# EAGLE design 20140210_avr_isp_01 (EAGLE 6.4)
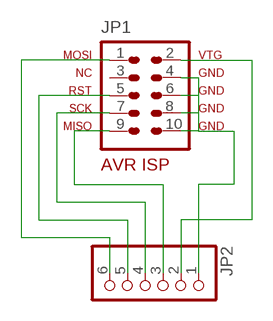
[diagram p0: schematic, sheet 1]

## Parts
JP1  AVR-ISP-10EDGE  [AVR-ISP-10-EDGE]
JP2  PINHD-1X6/90  [1X06/90]

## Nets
N$1: JP1.1 JP2.6
N$2: JP1.5 JP2.5
N$3: JP1.7 JP2.4
N$4: JP1.9 JP2.3
N$5: JP1.2 JP2.2
N$6: JP1.4 JP1.6 JP1.8 JP1.10 JP2.1
Unconnected: JP1.3

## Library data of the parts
JP1 = avr-4:AVR-ISP-10: AVR ISP-10 Serial Programming Header
JP2 = pinhead:PINHD-1X6: PIN HEADER

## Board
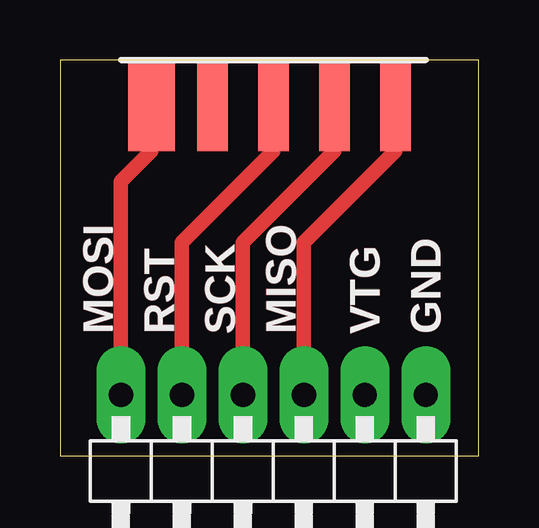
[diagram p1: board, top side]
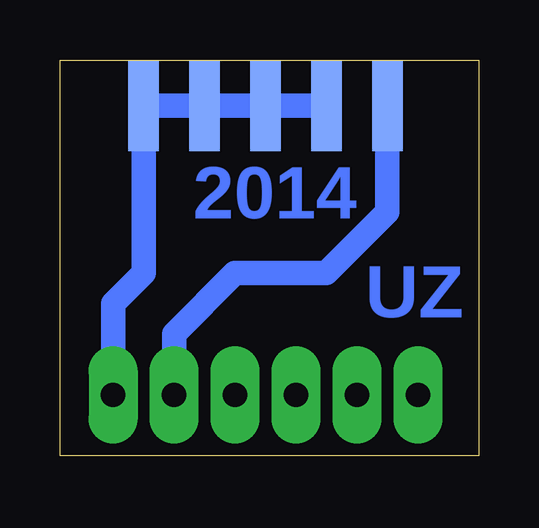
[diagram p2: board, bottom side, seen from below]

Size 17.45 x 16.5 mm. Coordinates in mm from the lower left corner, seen from the top.
Outline: 0,0 17.45,0 17.45,16.5 0,16.5 0,0
Copper layers (1*16): Top 0.035mm / dielectric 1.5mm / Bottom 0.035mm
Design rules "default *": minimum track width 10mil, minimum drill 24mil, track to track 8mil, track to pad 8mil, pad to pad 8mil, via to via 8mil, smd to smd 8mil, copper to edge 40mil, drill to drill 8mil, minimum pad ring 10mil, minimum via ring 8mil, stop-mask expansion 4mil, vias tented up to drill 0mil, thermal gap 10mil

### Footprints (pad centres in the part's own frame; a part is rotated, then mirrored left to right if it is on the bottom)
AVR-ISP-10-EDGE = smd 1.93 x 3.81: 1 -5.08,-1.905 | smd 1.27 x 3.81 bottom: 2 -5.08,-1.905; 4 -2.54,-1.905; 6 0,-1.905; 8 2.54,-1.905; 10 5.08,-1.905 | smd 1.27 x 3.81: 3 -2.54,-1.905; 5 0,-1.905; 7 2.54,-1.905; 9 5.08,-1.905
1X06/90 = drill 1.016 long: 1 -6.35,-3.81; 2 -3.81,-3.81; 3 -1.27,-3.81; 4 1.27,-3.81; 5 3.81,-3.81; 6 6.35,-3.81

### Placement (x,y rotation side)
JP1  8.89,16.51 0 top
JP2  8.89,-1.27 180 top

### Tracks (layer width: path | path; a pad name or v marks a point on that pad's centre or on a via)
N$1
  Top 0.61: JP1.1 3.81,12.7 2.54,11.43 JP2.6
N$2
  Top 0.61: JP1.5 8.89,12.7 5.08,8.89 JP2.5
N$3
  Top 0.61: JP1.7 11.43,12.7 7.62,8.89 JP2.4
N$4
  Top 0.61: JP1.9 13.97,12.7 10.16,8.89 JP2.3
N$5
  Bottom 1.016: JP1.2 3.81,10.16 6.35,7.62 10.16,7.62 12.7,5.08 JP2.2
N$6
  Bottom 1.016: JP1.4 JP1.6 JP1.8 JP1.10 13.97,7.62 15.24,6.35 JP2.1

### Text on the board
Top: MOSI | RST | SCK | MISO | VTG | GND
Bottom: 2014 | UZ
tPlace: MOSI | RST | SCK | MISO | VTG | GND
